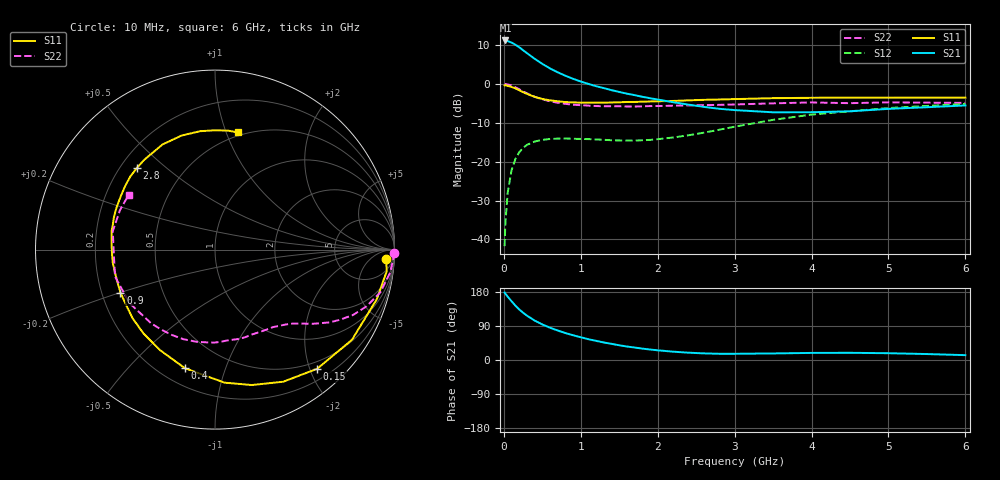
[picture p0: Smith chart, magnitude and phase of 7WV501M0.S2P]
! Infineon Technologies  Discrete & RF Semiconductors
! BFS17W
! Si NPN RF Bipolar Junction Transistor in SOT323
! VCE = 0.5 V  IC = 1 mA
! Common Emitter S-Parameters:  August  1999
# GHz  S  MA  R  50
!  f  S11  S21  S12  S22
! GHz  MAG  ANG  MAG  ANG  MAG  ANG  MAG  ANG
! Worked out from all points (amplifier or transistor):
!   36 points, 10 MHz to 6 GHz, reference 50 ohm
!   highest |S21| = 11.2 dB at 20 MHz (marker M1)
!   |S21| within 3 dB of that: start of sweep to 283 MHz
!   unconditionally stable (mu >= 1): 880.7 MHz to end of sweep
!   at 250 MHz: K = 0.31, MSG = 12.6 dB, |S12| = -16.5 dB
!   at 1.4 GHz: K = 1.43, MAG = 2.5 dB, |S12| = -14.5 dB
!   at 6 GHz: K = 1.16, MAG = -2.6 dB, |S12| = -5.2 dB
!   S11 on the Smith chart (normalised r, x): 10 MHz: 17, -21; 150 MHz: 0.38, -2.12; 400 MHz: 0.30, -0.73; 900 MHz: 0.28, -0.20; 2.8 GHz: 0.27, +0.40; 6 GHz: 0.47, +1.10
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0.01  0.9546 -3.3  3.587 178.2  0.0082 89.1  0.9984 -1.0
0.02  0.9647 -7.1  3.613 175.0  0.0162 86.8  0.9944 -3.1
0.05  0.9431 -17.0  3.545 167.1  0.0399 80.2  0.9841 -7.5
0.1  0.9137 -33.4  3.396 155.1  0.0774 69.8  0.9515 -14.5
0.15  0.8745 -49.4  3.189 143.5  0.108 60.6  0.9017 -20.5
0.2  0.8284 -62.7  2.956 133.5  0.1321 53.6  0.8514 -25.3
0.25  0.7819 -74.8  2.705 124.8  0.1501 46.9  0.7987 -29.3
0.3  0.7432 -85.9  2.485 117.1  0.1642 42.2  0.7567 -32.4
0.4  0.6817 -104.2  2.102 104.1  0.1814 34.1  0.6825 -37.3
0.5  0.6388 -118.5  1.807 93.9  0.1905 28.8  0.6328 -40.6
0.6  0.6141 -130.4  1.578 85.2  0.1956 25.1  0.5967 -43.7
0.7  0.5977 -140.2  1.409 77.8  0.1977 22.6  0.5721 -46.9
0.9  0.5787 -155.6  1.162 65.3  0.1971 19.3  0.5394 -53.2
1.1  0.572 -167.8  0.998 54.8  0.1948 18.5  0.5247 -60.0
1.6  0.5852 170.0  0.748 35.6  0.1868 23.0  0.5117 -78.7
2.2  0.6031 150.7  0.581 22.0  0.2045 35.1  0.524 -101.6
2.8  0.6296 133.6  0.478 16.4  0.2573 42.6  0.5372 -124.1
3.5  0.6547 116.5  0.431 17.3  0.3448 41.9  0.5619 -148.0
4  0.6621 106.4  0.432 18.7  0.4027 37.4  0.577 -164.9
4.5  0.6649 97.2  0.444 19.0  0.4441 32.2  0.5647 -179.3
5.5  0.6667 83.8  0.501 15.7  0.5204 22.4  0.5733 157.5
6  0.6657 78.9  0.528 12.8  0.5514 17.7  0.5697 147.4
